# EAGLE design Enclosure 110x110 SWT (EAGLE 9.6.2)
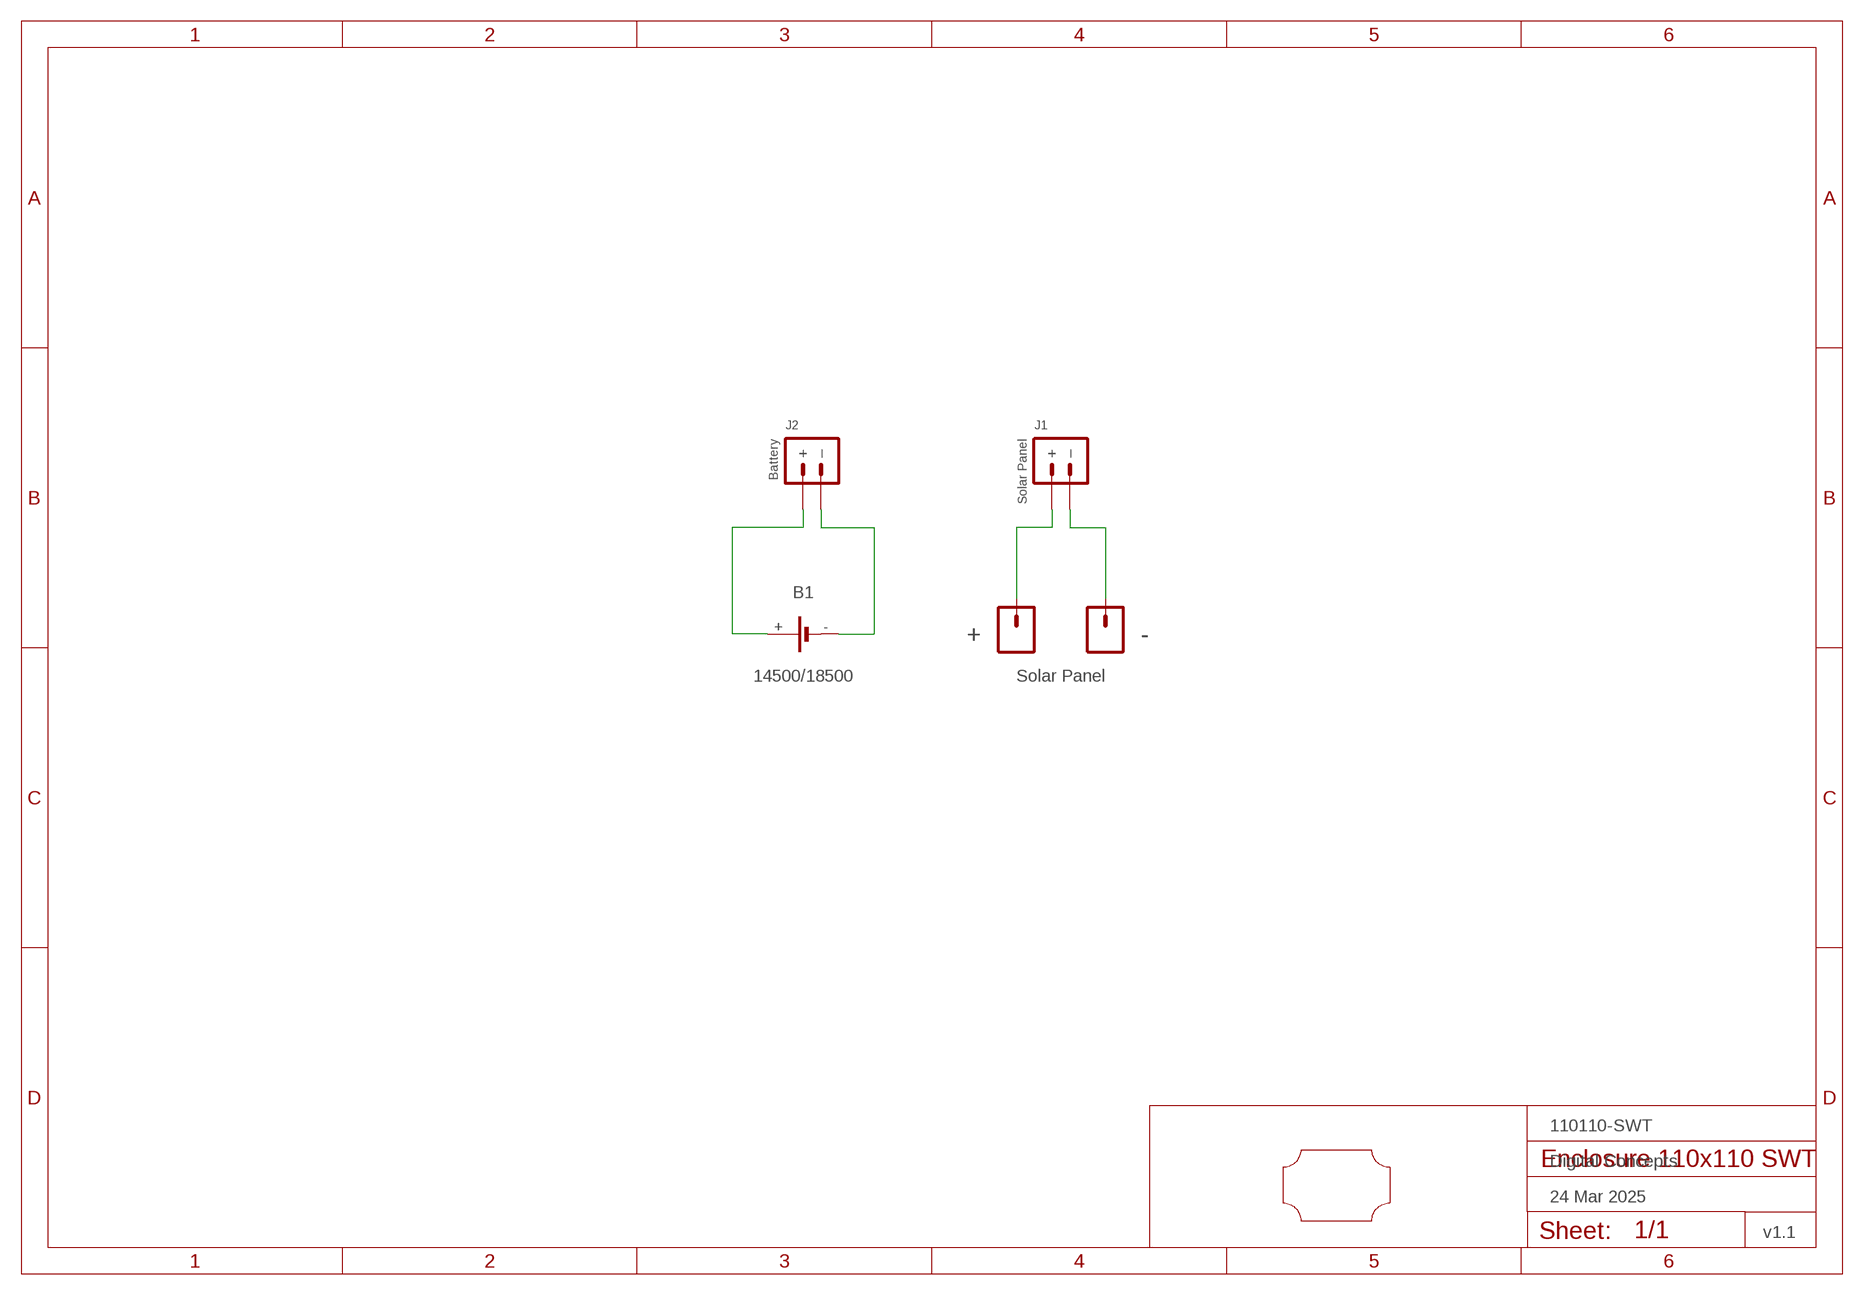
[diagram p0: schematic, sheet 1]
FRAME1 (FRAME-A4L-LOC): DATE: 24 Mar 2025; OWNER: Digital Concepts; TITLE: 110110-SWT; VERSION: v1.1

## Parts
+  PAD-SMD-GENERIC-SQUARE  [PAD-SMD-GENERIC]
-  PAD-SMD-GENERIC-SQUARE  [PAD-SMD-GENERIC]
B1  14500/18500  BATTERY-HOLDER-14500/18500  [BATTERY-14500/18500]
J1  Solar Panel  JST-PH2.0-2-HORIZONTAL-POWERJST-PTH-2  [JST-PH2.0-2-HORIZONTAL-POWER]
J2  Battery  JST-PH2.0-2-HORIZONTAL-POWERJST-PTH-2  [JST-PH2.0-2-HORIZONTAL-POWER]
U$1  PCB-OUTLINE-110X110  [PROTO-110X110-OUTLINE]

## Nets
N$1: B1.+ J2.+
N$2: B1.- J2.-(–)
N$3: +.P$1 J1.+
N$4: -.P$1 J1.-(–)

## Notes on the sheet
- Solar Panel

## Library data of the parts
+ - = digitalconcepts:PAD-SMD-GENERIC-SQUARE: SMD Pad—Square
B1 = digitalconcepts:BATTERY-HOLDER-14500/18500: 14500/18500 Battery Holder
J1 J2 = digitalconcepts:JST-PH2.0-2-HORIZONTAL-POWER: PH2.0 2P Right Angle PCB Connector; PROD_ID: CONN-09863; SKU: PRT-09914
U$1 = digitalconcepts:PCB-OUTLINE-110X110: PCB outline for 110 x 110 enclosure (100x80 max)

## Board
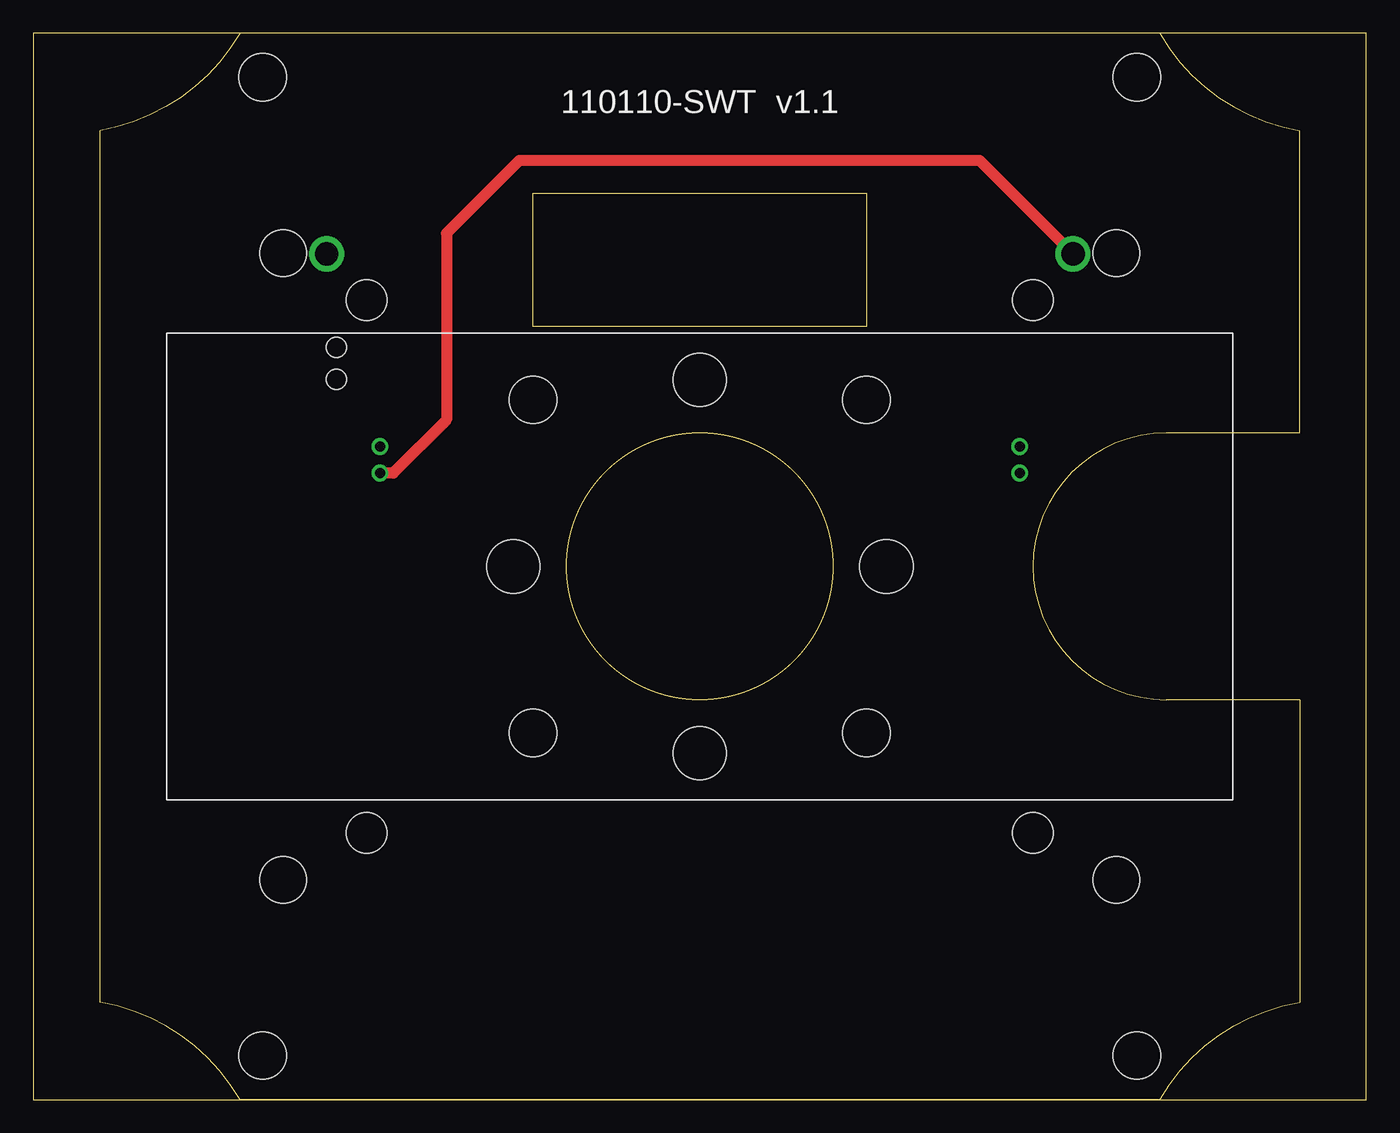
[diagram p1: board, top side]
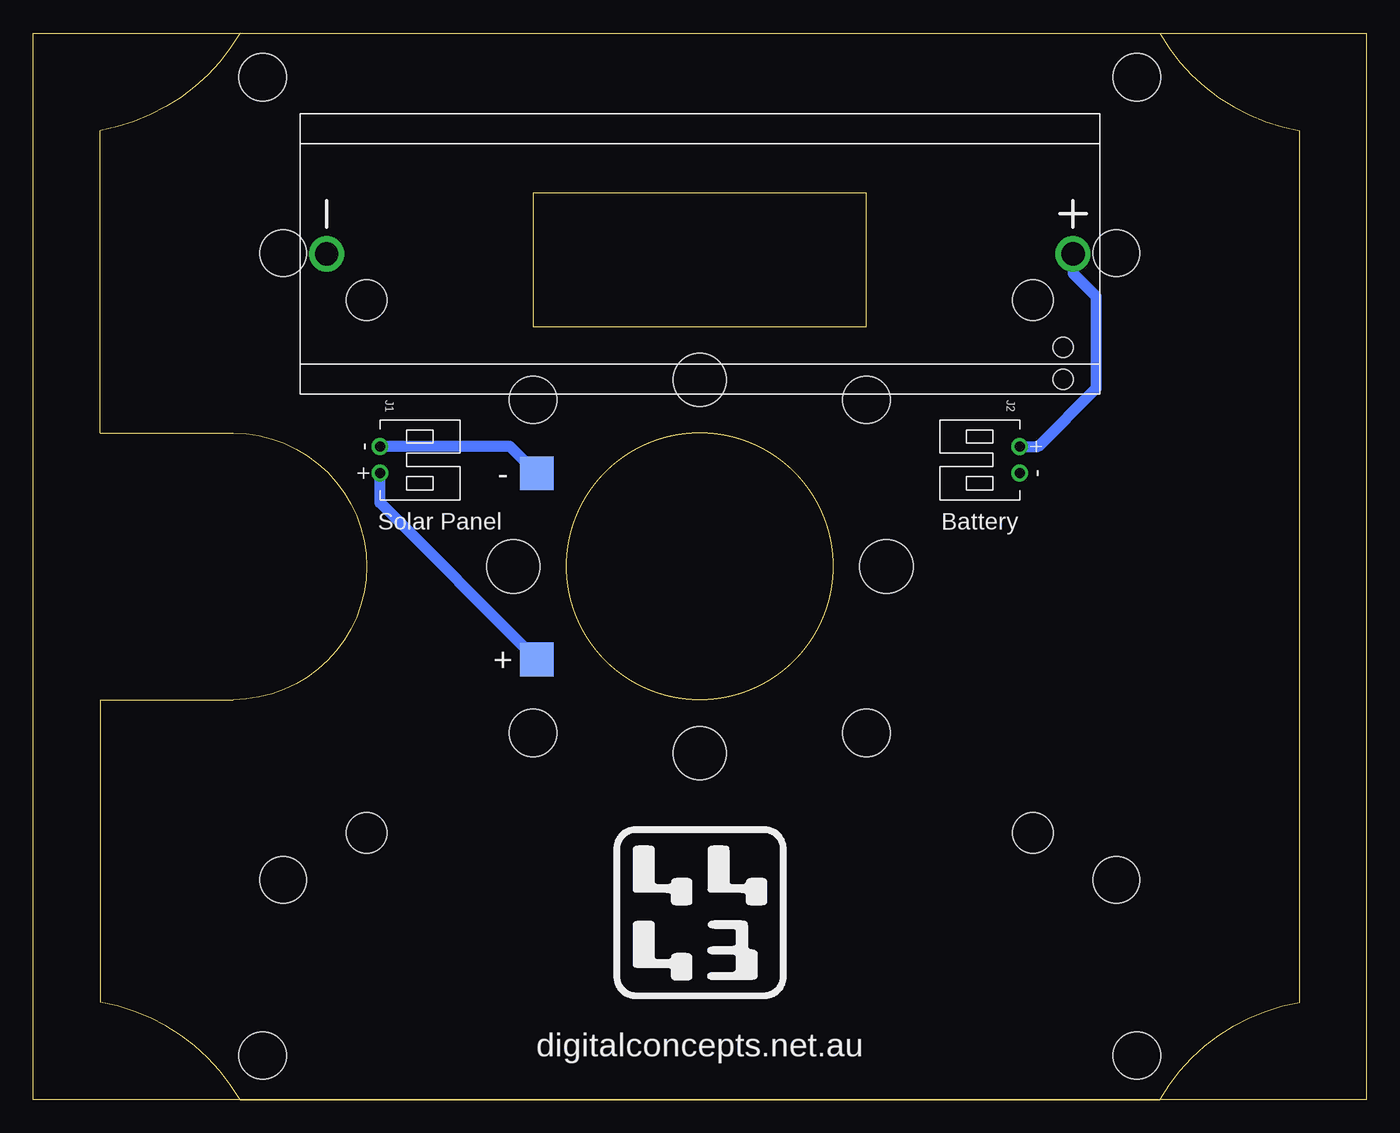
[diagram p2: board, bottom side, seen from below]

Size 100 x 80 mm. Coordinates in mm from the lower left corner, seen from the top.
Outline: 0,0 100,0 100,80 0,80 0,0
Outline: 37.5,68 62.5,68 62.5,58 37.5,58 37.5,68
Outline: circle at 50,40 radius 10
Copper layers (1*16): Top 0.035mm / dielectric 1.5mm / Bottom 0.035mm
Design rules "default *": minimum track width 6mil, minimum drill 0.35mm, track to track 6mil, track to pad 6mil, pad to pad 6mil, via to via 6mil, smd to smd 6mil, copper to edge 6mil, drill to drill 6mil, minimum pad ring 10mil, minimum via ring 8mil, stop-mask expansion 4mil, vias tented up to drill 0mil, thermal gap 10mil

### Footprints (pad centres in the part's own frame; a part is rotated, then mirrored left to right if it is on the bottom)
PAD-SMD-GENERIC = smd 2.54 x 2.54: P$1 0,0
BATTERY-14500/18500 = drill 1.75: + -28,0; - 28,0 | hole 1.524: -27.25,9.4; -27.25,7
JST-PH2.0-2-HORIZONTAL-POWER = drill 0.75: + 1,0; - -1,0
PROTO-110X110-OUTLINE = hole 3.556: -12.5,12.5; -12.5,-12.5; 12.5,-12.5; 12.5,12.5; -32.8,36.7; 32.8,36.7; 32.8,-36.7; -32.8,-36.7 | hole 3.048: -24.994,19.99; 24.994,19.99; 24.994,-19.99; -24.994,-19.99 | hole 3.5: -31.25,23.5; 31.25,23.5; 31.25,-23.5; -31.25,-23.5 | hole 4: 0,14; 0,-14; 14,0; -14,0

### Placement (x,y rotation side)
+  62.23,33.02 0 bottom
-  62.23,46.99 0 bottom
B1  50,63.45 180 bottom
J1  74,48 270 bottom
J2  26,48 90 bottom
U$1  50,40 0 top

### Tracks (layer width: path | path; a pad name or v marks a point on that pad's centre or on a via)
N$1
  Bottom 0.813: J2.+ 24.6,49 20.27,53.33 20.27,60.27 22,62 B1.+
N$2
  Top 0.813: B1.- 71,70.45 36.45,70.45 31,65 31,51 27,47 J2.-
N$3
  Bottom 0.813: +.P$1 74,44.79 J1.+
N$4
  Bottom 0.813: -.P$1 64.24,49 J1.-

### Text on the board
tPlace: 110110-SWT v1.1
bPlace: digitalconcepts.net.au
